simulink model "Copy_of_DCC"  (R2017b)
settings: Solver=FixedStepDiscrete  StartTime=0.0  StopTime=10.0  FixedStep=0.01  RelTol=1e-3  EnableMultiTasking=on
undefined symbols (not defined in the file): ASWTYPE_FALSE, ASWTYPE_TRUE, CbDCC_BMTMsgCmd_flg, CbDCC_BMVMsgCmd_flg, CbDCC_BSPMsgCmd_flg, CcDCC_BSTSendTi_ms, CcDCC_BulkSOC_pct, CcDCC_CCSTout_ms, CcDCC_CellTempFilterAvg_numb, CcDCC_ChrgCrnt0HysVolt_mV, CcDCC_ChrgFinOverTi_ms, CcDCC_ChrgMaxPackVoltLimt_V, CcDCC_ChrgSt2StepChrgTime_ms, CcDCC_ChrgStCutoffTime_ms, CcDCC_ChrgStFullChrgCrnt_A, CcDCC_CMLTout_ms, CcDCC_CommToutOverTi_ms, CcDCC_CRMAATout_ms, CcDCC_CRMCHMTout_ms, CcDCC_CRMTout_ms, CcDCC_CROAATout_ms, CcDCC_CROTout_ms, CcDCC_CSDTout_ms, CcDCC_CSTTout_ms, CcDCC_DC12VUnonnectTi_ms, CcDCC_DCChrgDispSOCPrmt_pct, CcDCC_DCChrgMismatch_ms, CcDCC_DCChrgPermitCfg_ms, CcDCC_DCChrgPrmtFltLvl_numb, CcDCC_DCChrgPrmtStop_ms, CcDCC_DCChrgStepCurr_A, CcDCC_DCChrgStop_ms, CcDCC_DCCrntUnctrolTi_ms, CcDCC_DCFullChrgHysVolt_mV, CcDCC_DCFullStepChrgTi1_ms, CcDCC_DCFullStepChrgTi2_ms, CcDCC_DCMaxChrgCurr_A, CcDCC_DCStepChrgWaitTime_ms, CcDCC_DCStop2DefaultTi_ms, CcDCC_DefaultWaitTi_ms, CcDCC_DiffDCChrgCrnt_A, CcDCC_DiffDCChrgCrntTi_ms, CcDCC_HeatChrgCrnt0Time_ms, CcDCC_HeatChrgCrnt1Time_ms, CcDCC_IsoDisableDelay_ms, CcDCC_MaxPackVoltLimt_V, CcDCC_SafeCur_A, CcDCC_StartChrgHysVolt_mV, CcDCC_StartDCChrgCellTemp_C, CcDCC_StepChrgCutoffTi_ms, CcDCC_StepChrgFullChrgCrnt_A, CcDCC_ToutDelay_ms, CcDCC_VehSpdFld_kmh, DCC_CONST0_NUMB, DCC_CONST1000_NUMB, DCC_CONST170_NUMB, DCC_RUNTIME_MS, Enum_BTMHeatReq, Enum_CTCCtrCtlConnMode, Enum_CTCCtrCtlState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
libraries: AIWAYS_Powertrain_BMS_lib x82
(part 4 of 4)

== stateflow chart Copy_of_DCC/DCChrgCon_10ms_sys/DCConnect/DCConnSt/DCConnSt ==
  state Default
    en:
    GeDCC_DCConnSt_enum = Enum_DCCDCConnSt.Enum_DCCDCConnSt_Default;
    GbDCC_BHMMsgCmd_flg = ASWTYPE_FALSE;
    GbDCC_BRMMsgCmd_flg = ASWTYPE_FALSE;
    GbDCC_BCPMsgCmd_flg = ASWTYPE_FALSE;
    GbDCC_BROMsgCmd_flg = ASWTYPE_FALSE;
    GbDCC_BCLMsgCmd_flg = ASWTYPE_FALSE;
    GbDCC_BCSMsgCmd_flg = ASWTYPE_FALSE;
    GbDCC_BSMMsgCmd_flg = ASWTYPE_FALSE;
    GbDCC_BMVMsgCmd_flg = ASWTYPE_FALSE;
    GbDCC_BMTMsgCmd_flg = ASWTYPE_FALSE;
    GbDCC_BSPMsgCmd_flg = ASWTYPE_FALSE;
    GbDCC_BSTMsgCmd_flg = ASWTYPE_FALSE;
    GbDCC_BSDMsgCmd_flg = ASWTYPE_FALSE;
    GbDCC_CRM00Tout_flg = ASWTYPE_FALSE;
    GbDCC_CRMAATout_flg = ASWTYPE_FALSE;
    GbDCC_CROTout_flg = ASWTYPE_FALSE;
    GbDCC_CMLTout_flg = ASWTYPE_FALSE;
    GbDCC_CROAATout_flg = ASWTYPE_FALSE;
    GbDCC_CCSTout_flg = ASWTYPE_FALSE;
    GbDCC_CSTTout_flg = ASWTYPE_FALSE;
    GbDCC_CSDTout_flg = ASWTYPE_FALSE;
    GbDCC_DCChrgRqst_flg = ASWTYPE_FALSE;
  state HandShake
    en:
    GeDCC_DCConnSt_enum = Enum_DCCDCConnSt.Enum_DCCDCConnSt_HandShake;
    GbDCC_BHMMsgCmd_flg = GbGDP_CHMRecOnce_flg;
    GbDCC_CRM00Tout_flg = CRM00Timeout(GbGDP_CHMRecOnce_flg);
    du:
    GbDCC_BHMMsgCmd_flg = GbGDP_CHMRecOnce_flg;
    GbDCC_CRM00Tout_flg = CRM00Timeout(GbGDP_CHMRecOnce_flg);
    ex:
    GbDCC_BHMMsgCmd_flg = ASWTYPE_FALSE;
    state GbDCC_CRM00Tout_flg = CRM00Timeout(GbGDP_CHMRecOnce_flg) [function]
  state ID
    en:
    GeDCC_DCConnSt_enum = Enum_DCCDCConnSt.Enum_DCCDCConnSt_ID;
    GbDCC_BRMMsgCmd_flg = ASWTYPE_TRUE;
    GbDCC_CRMAATout_flg = CRMAATimeout(GbGDP_CRMRecOnce_flg,GcGDP_CRMChrgrAck_numb)
    du:
    GbDCC_CRMAATout_flg = CRMAATimeout(GbGDP_CRMRecOnce_flg,GcGDP_CRMChrgrAck_numb)
    ex:
    GbDCC_BRMMsgCmd_flg = ASWTYPE_FALSE;
    state GbDCC_CRMAATout_flg = CRMAATimeout(GbGDP_CRMRecOnce_flg,GcGDP_CRMChrgrAck_numb) [function]
  state CFG
    en:
    GeDCC_DCConnSt_enum = Enum_DCCDCConnSt.Enum_DCCDCConnSt_CFG;
    GbDCC_BCPMsgCmd_flg = ASWTYPE_TRUE;
    GbDCC_CROTout_flg = CRO00Timeout(GbGDP_CRORecOnce_flg,GbDCC_BROMsgCmd_flg,GcGDP_CROChrgrRdy_numb,GcDCS_2829Da_numb);
    GbDCC_CMLTout_flg = CMLTimeout(GbGDP_CMLRecOnce_flg);
    GbDCC_CROAATout_flg = CROAATimeout(GbGDP_CRORecOnce_flg,GbDCC_BROMsgCmd_flg,GcGDP_CROChrgrRdy_numb,GcDCS_2829Da_numb);
    GbDCC_DCChrgRqst_flg = GbGDP_CMLRecOnce_flg;
    du:
    GbDCC_BCPMsgCmd_flg = (GbGDP_CMLRecOnce_flg==ASWTYPE_FALSE);
    GbDCC_BROMsgCmd_flg = GbGDP_CMLRecOnce_flg;
    GbDCC_CROTout_flg = CRO00Timeout(GbGDP_CRORecOnce_flg,GbDCC_BROMsgCmd_flg,GcGDP_CROChrgrRdy_numb,GcDCS_2829Da_numb);
    GbDCC_CMLTout_flg = CMLTimeout(GbGDP_CMLRecOnce_flg);
    GbDCC_CROAATout_flg = CROAATimeout(GbGDP_CRORecOnce_flg,GbDCC_BROMsgCmd_flg,GcGDP_CROChrgrRdy_numb,GcDCS_2829Da_numb);
    GbDCC_DCChrgRqst_flg = GbGDP_CMLRecOnce_flg;
    ex:
    GbDCC_BCPMsgCmd_flg = ASWTYPE_FALSE;
    GbDCC_BROMsgCmd_flg = ASWTYPE_FALSE;
    state GbDCC_CMLTout_flg = CMLTimeout(GbGDP_CMLRecOnce_flg) [function]
    state GbDCC_CROTout_flg = CRO00Timeout(GbGDP_CRORecOnce_flg,GbDCC_BROMsgCmd_flg,GcGDP_CROChrgrRdy_numb,GcDCS_2829Da_numb) [function]
    state GbDCC_CROAATout_flg = CROAATimeout(GbGDP_CRORecOnce_flg,GbDCC_BROMsgCmd_flg,GcGDP_CROChrgrRdy_numb,GcDCS_2829Da_numb) [function]
  state CommTout
    en:
    GeDCC_DCConnSt_enum=Enum_DCCDCConnSt.Enum_DCCDCConnSt_CommTout;
    GbDCC_BEMMsgCmd_flg = (GbGDP_CEMRecOnce_flg==ASWTYPE_FALSE);
    GbDCC_DCChrgRqst_flg = ASWTYPE_FALSE;
    du:
    GbDCC_BEMMsgCmd_flg = (GbGDP_CEMRecOnce_flg==ASWTYPE_FALSE);
    ex:
    GbDCC_BEMMsgCmd_flg = ASWTYPE_FALSE;
  state Chrging
    en:
    GeDCC_DCConnSt_enum = Enum_DCCDCConnSt.Enum_DCCDCConnSt_Chrging;
    GbDCC_BCLMsgCmd_flg = ASWTYPE_TRUE;
    GbDCC_BCSMsgCmd_flg = ASWTYPE_TRUE;
    GbDCC_CCSTout_flg = CCSTimeout(GbGDP_CCSMsgUpd_flg);
    GbDCC_DCChrgRqst_flg = ASWTYPE_TRUE;
    du:
    GbDCC_BSMMsgCmd_flg = GbGDP_CCSRecOnce_flg;
    GbDCC_BMTMsgCmd_flg = (GbGDP_CCSRecOnce_flg&&CbDCC_BMTMsgCmd_flg);
    GbDCC_BMVMsgCmd_flg = (GbGDP_CCSRecOnce_flg&&CbDCC_BMVMsgCmd_flg);
    GbDCC_BSPMsgCmd_flg = (GbGDP_CCSRecOnce_flg&&CbDCC_BSPMsgCmd_flg);
    GbDCC_CCSTout_flg = CCSTimeout(GbGDP_CCSMsgUpd_flg)
    ex:
    GbDCC_BCLMsgCmd_flg = ASWTYPE_FALSE;
    GbDCC_BCSMsgCmd_flg = ASWTYPE_FALSE;
    GbDCC_BSMMsgCmd_flg = ASWTYPE_FALSE;
    GbDCC_BMVMsgCmd_flg = ASWTYPE_FALSE;
    GbDCC_BMTMsgCmd_flg = ASWTYPE_FALSE;
    GbDCC_BSPMsgCmd_flg = ASWTYPE_FALSE;
    state GbDCC_CCSTout_flg = CCSTimeout(GbGDP_CCSMsgUpd_flg) [function]
  state ChrgFin
    en:
    GeDCC_DCConnSt_enum = Enum_DCCDCConnSt.Enum_DCCDCConnSt_ChrgFin;
    GbDCC_BSTMsgCmd_flg = ASWTYPE_TRUE;
    GbDCC_CSTTout_flg = CSTTimeout(GbGDP_CSTRecOnce_flg);
    GbDCC_CSDTout_flg = CSDTimeout(GbGDP_CSDRecOnce_flg);
    GbDCC_DCChrgRqst_flg = ASWTYPE_FALSE;
    du:
    GbDCC_CSTTout_flg = CSTTimeout(GbGDP_CSTRecOnce_flg);
    GbDCC_CSDTout_flg = CSDTimeout(GbGDP_CSDRecOnce_flg);
    GbDCC_BSDMsgCmd_flg = BSDMsgCmd(GbGDP_CSTRecOnce_flg,GbDCC_CSTTout_flg);
    GbDCC_BSTMsgCmd_flg = (ASWTYPE_FALSE == GbDCC_BSDMsgCmd_flg);
    ex:
    GbDCC_BSTMsgCmd_flg = ASWTYPE_FALSE;
    GbDCC_BSDMsgCmd_flg = ASWTYPE_FALSE;
    state GbDCC_CSTTout_flg = CSTTimeout(GbGDP_CSTRecOnce_flg) [function]
    state GbDCC_CSDTout_flg = CSDTimeout(GbGDP_CSDRecOnce_flg) [function]
    state GbDCC_BSDMsgCmd_flg = BSDMsgCmd(GbGDP_CSTRecOnce_flg,GbDCC_CSTTout_flg) [function]
  (default) -> Default
  (junction 323) -> Default
  (junction 331) -> Default
  (junction 325) -> (junction 323)
  CommTout -> (junction 331) : [ASWTYPE_TRUE == LbDCC_DCCommTout2Default_flg]
  (junction 434) -> Default
  (junction 435) -> (junction 434) : [ASWTYPE_TRUE == LbDCC_DCID2Default_flg]
  (junction 431) -> Default
  (junction 429) -> (junction 431) : [ASWTYPE_TRUE == LbDCC_DCHandShake2Default_flg]
  Default -> HandShake : [ASWTYPE_TRUE == LbDCC_DCDefault2Handshake_flg]
  HandShake -> (junction 333) : [(ASWTYPE_TRUE == GbDCC_CRM00Tout_flg)||(ASWTYPE_TRUE == GbGDP_CEMRecOnce_flg)]
  (junction 333) -> CommTout
  HandShake -> (junction 429)
  HandShake -> ID : [(ASWTYPE_TRUE == GbGDP_CRMRecOnce_flg)&&... (DCC_CONST0_NUMB == GcGDP_CRMChrgrAck_numb)]
  ID -> (junction 335) : [(ASWTYPE_TRUE == GbDCC_CRMAATout_flg)||(ASWTYPE_TRUE == GbGDP_CEMRecOnce_flg)]
  (junction 335) -> CommTout
  ID -> (junction 435)
  ID -> CFG : [(ASWTYPE_TRUE == GbGDP_CRMRecOnce_flg)&&... (DCC_CONST170_NUMB == GcGDP_CRMChrgrAck_numb)]
  CFG -> (junction 417) : [ASWTYPE_TRUE == LbDCC_DCCFG2ChrgFinish_flg]
  (junction 417) -> (junction 419)
  CFG -> CommTout : [(ASWTYPE_TRUE == GbDCC_CROTout_flg)||... (ASWTYPE_TRUE == GbGDP_CEMRecOnce_flg)||... (ASWTYPE_TRUE == GbDCC_CROAATout_flg)||... (ASWTYPE_TRUE == GbDCC_CMLTout_flg)]
  (junction 329) -> CommTout
  (junction 327) -> CommTout
  CFG -> Chrging : [(ASWTYPE_TRUE == GbGDP_CRORecOnce_flg)&&... (DCC_CONST170_NUMB == GcGDP_CROChrgrRdy_numb)]
  Chrging -> (junction 329) : [(ASWTYPE_TRUE == GbDCC_CCSTout_flg)||(ASWTYPE_TRUE == GbGDP_CEMRecOnce_flg)]
  Chrging -> ChrgFin : [ASWTYPE_TRUE == LbDCC_DCChrging2ChrgFin_flg]
  (junction 419) -> ChrgFin
  ChrgFin -> (junction 327) : [(ASWTYPE_TRUE == GbDCC_CSTTout_flg)||... (ASWTYPE_TRUE == GbDCC_CSDTout_flg)||... (ASWTYPE_TRUE == GbGDP_CEMRecOnce_flg)]
  ChrgFin -> (junction 325) : [((ASWTYPE_TRUE == GbGDP_CRMMsgUpd_flg) || (ASWTYPE_FALSE == GbLDP_DC12VSply_flg))...  &&(GeCTC_CtrCtlConnMode_enum != Enum_CTCCtrCtlConnMode.Enum_CTCCtrCtlConnMode_DCChrg)]
  data: GbDCC_CRM00Tout_flg function_output boolean; GbGDP_CHMRecOnce_flg function_input boolean; GbGDP_CRMRecOnce_flg function_input boolean; GcGDP_CRMChrgrAck_numb function_input uint8; GbDCC_CRMAATout_flg function_output boolean; GbGDP_CMLRecOnce_flg function_input boolean; GbDCC_CMLTout_flg function_output boolean; GbGDP_CRORecOnce_flg function_input boolean; GbDCC_BROMsgCmd_flg function_input boolean; GcGDP_CROChrgrRdy_numb function_input uint8; GbDCC_CROTout_flg function_output boolean; GcDCS_2829Da_numb function_input uint8; GbGDP_CRORecOnce_flg function_input boolean; GbDCC_BROMsgCmd_flg function_input boolean; GbDCC_CROAATout_flg function_output boolean; GcGDP_CROChrgrRdy_numb function_input uint8; GcDCS_2829Da_numb function_input uint8; GbGDP_CCSMsgUpd_flg function_input boolean; GbDCC_CCSTout_flg function_output boolean; GbGDP_CSTRecOnce_flg function_input boolean; GbDCC_CSTTout_flg function_output boolean; GbGDP_CSDRecOnce_flg function_input boolean; GbDCC_CSDTout_flg function_output boolean; GbGDP_CSTRecOnce_flg function_input boolean; GbDCC_CSTTout_flg function_input; GbDCC_BSDMsgCmd_flg function_output boolean; GbGDP_CHMRecOnce_flg input; GbGDP_CMLRecOnce_flg input; GbGDP_CCSRecOnce_flg input; GbGDP_CEMRecOnce_flg input; GbGDP_CRMRecOnce_flg input; GbGDP_CRMMsgUpd_flg input; GbGDP_CRORecOnce_flg input; GbGDP_CSDRecOnce_flg input; GbGDP_CSTRecOnce_flg input; GcGDP_CRMChrgrAck_numb input; GcGDP_CROChrgrRdy_numb input; GcDCS_2829Da_numb input; GbLDP_DC12VSply_flg input; ASWTYPE_TRUE parameter; ASWTYPE_FALSE parameter; GeDCC_DCConnSt_enum output; GbDCC_BHMMsgCmd_flg output; GbDCC_BRMMsgCmd_flg output; GbDCC_BCPMsgCmd_flg output; GbDCC_BROMsgCmd_flg output; GbDCC_BCLMsgCmd_flg output; GbDCC_BCSMsgCmd_flg output; GbDCC_BSMMsgCmd_flg output; GbDCC_BMVMsgCmd_flg output; GbDCC_BMTMsgCmd_flg output; GbDCC_BSPMsgCmd_flg output; GbDCC_BSTMsgCmd_flg output; GbDCC_BSDMsgCmd_flg output; GbDCC_BEMMsgCmd_flg output; LbDCC_DCDefault2Handshake_flg input; LbDCC_DCHandShake2Default_flg input; LbDCC_DCID2Default_flg input; LbDCC_DCCFG2ChrgFinish_flg input; LbDCC_DCChrging2ChrgFin_flg input; LbDCC_DCCommTout2Default_flg input; DCC_CONST170_NUMB parameter; GbDCC_CRM00Tout_flg output; GbDCC_CRMAATout_flg output; GbDCC_CROTout_flg output; GbDCC_CROAATout_flg output; GbDCC_CMLTout_flg output; GbDCC_CCSTout_flg output; GbDCC_CSTTout_flg output; GbDCC_CSDTout_flg output; CbDCC_BMTMsgCmd_flg parameter; CbDCC_BMVMsgCmd_flg parameter; CbDCC_BSPMsgCmd_flg parameter; GbGDP_CCSMsgUpd_flg input; DCC_CONST0_NUMB parameter; GeCTC_CtrCtlConnMode_enum input; GbDCC_DCChrgRqst_flg output

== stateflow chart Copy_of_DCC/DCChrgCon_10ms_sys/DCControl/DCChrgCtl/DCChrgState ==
  state DCC_DCDefault
    en:
    GeDCC_DCChrgState_enum = Enum_DCCDCChrgState.Enum_DCCDCChrgState_Default;
    GcDCC_DCChrgVoltRqst_V = GcHDP_PackVolt_V;
    LcDCC_DCChrgCurrRqst_A = DCC_CONST0_NUMB;
    GbDCC_DCChrgFinish_flg = ASWTYPE_FALSE;
  state DCC_DCChrg
    en:
    GeDCC_DCChrgState_enum = Enum_DCCDCChrgState.Enum_DCCDCChrgState_Chrg;
    GcDCC_DCChrgVoltRqst_V = CcDCC_ChrgMaxPackVoltLimt_V;
    LcDCC_DCChrgCurrRqst_A = GcSOP_MaxChrgCurr_A;
    du:
    LcDCC_DCChrgCurrRqst_A = GcSOP_MaxChrgCurr_A;
    ex:
    GbDCC_DCChrgFinish_flg = LbDCC_FinishInChrgSt_flg;
  state DCC_DCStop
    en:
    GeDCC_DCChrgState_enum = Enum_DCCDCChrgState.Enum_DCCDCChrgState_Stop;
    GcDCC_DCChrgVoltRqst_V = CcDCC_ChrgMaxPackVoltLimt_V;
    LcDCC_DCChrgCurrRqst_A = DCC_CONST0_NUMB;
  state DCC_DCStepChrg
    en:
    GeDCC_DCChrgState_enum = Enum_DCCDCChrgState.Enum_DCCDCChrgState_StepChrg;
    GcDCC_DCChrgVoltRqst_V = CcDCC_ChrgMaxPackVoltLimt_V;
    du:
    LcDCC_DCChrgCurrRqst_A = LcDCC_StepChrgCrntReq_A;
    ex:
    GbDCC_DCChrgFinish_flg = LbDCC_FinishInStepChrg_flg;
  (default) -> DCC_DCDefault
  DCC_DCStop -> DCC_DCDefault : [ASWTYPE_TRUE == LbDCC_Stop2Default_flg]
  DCC_DCDefault -> DCC_DCChrg : [ASWTYPE_TRUE == LbDCC_ChrgStateDef2Chrg_flg]
  DCC_DCChrg -> DCC_DCStop : [ASWTYPE_TRUE == LbDCC_ChrgSt2Stop_flg]
  DCC_DCStepChrg -> DCC_DCStop : [ASWTYPE_TRUE== LbDCC_StepChrg2Stop_flg]
  DCC_DCChrg -> DCC_DCStepChrg : [ASWTYPE_TRUE == LbDCC_ChrgSt2StepChrg_flg]
  data: GeDCC_DCChrgState_enum output; LcDCC_DCChrgCurrRqst_A output; GcDCC_DCChrgVoltRqst_V output; LbDCC_ChrgStateDef2Chrg_flg input; CcDCC_ChrgMaxPackVoltLimt_V parameter; DCC_CONST0_NUMB parameter; LbDCC_ChrgSt2StepChrg_flg input; LbDCC_ChrgSt2Stop_flg input; LbDCC_FinishInChrgSt_flg input; LcDCC_StepChrgCrntReq_A input; LbDCC_StepChrg2Stop_flg input; LbDCC_FinishInStepChrg_flg input; ASWTYPE_TRUE parameter; GcHDP_PackVolt_V input; GcSOP_MaxChrgCurr_A input; GbDCC_DCChrgFinish_flg output; LbDCC_Stop2Default_flg input; ASWTYPE_FALSE parameter

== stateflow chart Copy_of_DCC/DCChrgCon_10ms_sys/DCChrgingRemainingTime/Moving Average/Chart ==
  (default) -> (junction 16)
  (junction 16) -> (junction 17) : [R]
  (junction 17) -> (junction 22) : {count = 0;...  sum = 0;...  buffer = 0;...  average = 0;...  index = 0;}
  (junction 16) -> (junction 18)
  (junction 18) -> (junction 19) : [count >= BufferSize]
  (junction 18) -> (junction 21) : {count = count +1;}
  (junction 19) -> (junction 20) : {sum = sum - buffer[index];}
  (junction 20) -> (junction 21)
  (junction 21) -> (junction 25) : {sum = sum + u;... buffer[index] =u;... average = sum/count;}
  (junction 25) -> (junction 24) : [index >= BufferSize-1]
  (junction 25) -> (junction 26) : {index = index+1;}
  (junction 24) -> (junction 27) : {index = 0;}
  (junction 27) -> (junction 26)
  (junction 22) -> (junction 27)
  (junction 26) -> (junction 23) : {Y=average;}
  data: count local uint16 [0..500]; buffer local single; u input single; index local uint16 [0..499]; R input boolean; sum local single; BufferSize parameter uint16 [1..500]; Y output single; average local single

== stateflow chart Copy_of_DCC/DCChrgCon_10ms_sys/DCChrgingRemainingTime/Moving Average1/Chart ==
  (default) -> (junction 16)
  (junction 16) -> (junction 17) : [R]
  (junction 17) -> (junction 22) : {count = 0;...  sum = 0;...  buffer = 0;...  average = 0;...  index = 0;}
  (junction 16) -> (junction 18)
  (junction 18) -> (junction 19) : [count >= BufferSize]
  (junction 18) -> (junction 21) : {count = count +1;}
  (junction 19) -> (junction 20) : {sum = sum - buffer[index];}
  (junction 20) -> (junction 21)
  (junction 21) -> (junction 25) : {sum = sum + u;... buffer[index] =u;... average = sum/count;}
  (junction 25) -> (junction 24) : [index >= BufferSize-1]
  (junction 25) -> (junction 26) : {index = index+1;}
  (junction 24) -> (junction 27) : {index = 0;}
  (junction 27) -> (junction 26)
  (junction 22) -> (junction 27)
  (junction 26) -> (junction 23) : {Y=average;}
  data: count local uint16 [0..500]; buffer local single; u input single; index local uint16 [0..499]; R input boolean; sum local single; BufferSize parameter uint16 [1..500]; Y output single; average local single
